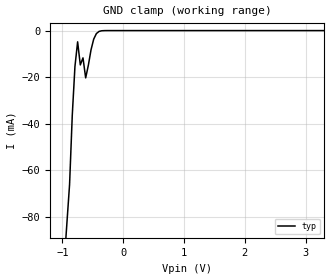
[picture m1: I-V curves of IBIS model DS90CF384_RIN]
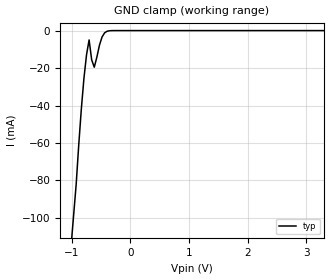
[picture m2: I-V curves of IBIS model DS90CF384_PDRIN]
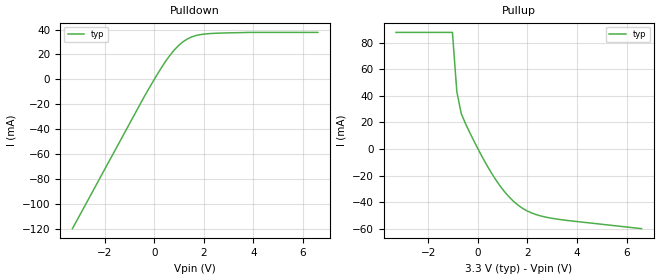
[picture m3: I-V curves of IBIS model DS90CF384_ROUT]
|   National Semiconductor Corporation
|   Interface Products Group
|   IBIS Model of 3.3V FPD-Link Receiver
|   56L TSSOP
[IBIS Ver]   2.1
[File name]   90cf384.ibs
[File Rev]   1.0
[Date]   7/10/98
[Source]   File originated at National Semiconductor Corporation.
   Interface Group/Analog Division. All data based on
   Empirical Measurements(Bench).
[Notes]   File created by SBH.
[Disclaimer]
(C) Copyright National Semiconductor Corporation 1994
   All rights reserved
   National Semiconductor Corporation hereby grants
the user of this IBIS model a non-exclusive, nontransferable
license to use this IBIS model under the following terms.
Before using this IBIS model, the user should read this
license.  If the user does not accept these terms,  the
IBIS model should be returned to National within 30 days.
   The user is granted this license only to use the
IBIS model and is not granted rights to sell, load, rent,
lease or license the IBIS model in whole or in part, or in
modified form to anyone other than user. User may modify
the IBIS model to suit its specific applications but rights
to derivative works and such modifications shall belong to
National.
   This IBIS model is provided on an "AS IS" basis and
National makes absolutely no warranty with respect to the
information contained herein.NATIONAL DISCLAIMS AND CUSTOMER
WAIVES ALL WARRANTIES, EXPRESS OR IMPLIED, INCLUDING
WARRANTIES OF MERCHANTABILITY OR FITNESS FOR A PARTICULAR
PURPOSE. The entire risk as to quality and performance is
with the Customer. ACCORDINGLY, IN NO EVENT SHALL THE
COMPANY BE LIABLE FOR ANY DAMAGES, WHETHER IN CONTRACT OR
TORT,INCLUDING ANY LOST PROFITS OR OTHER INCIDENTAL,
CONSEQUENTIAL, EXEMPLARY, OR PUNITIVE DAMAGES ARISING OUT
OF THE USE OR APPLICATION OF THE IBIS model provided in
this package.Further, National reserves the right to make
changes without notice to any product herein to improve
reliability, function, or design. National does not convey
any license under patent rights or any other intellectual
property rights, including those of third parties.
   National is not obligated to provide maintenance or support
for the licensed IBIS model.
Contact National at ATTN:INTERFACE APPLICATIONS/IBIS MODELS.
2900 Semiconductor Drive, M/S A2595, Santa Clara, CA 95052-8090
[Copyright]   Copyright 1994, National Semiconductor, All Rights Reserved
[Component]   DS90CF384MTD
[Manufacturer]  National Semiconductor Corp
[Package]
|   typ   min   max
R_pkg   35.0m   NA   NA
L_pkg   4.31nH   NA   NA
C_pkg   0.70pF   NA   NA
[Pin]  signal_name   model_name   R_pin   L_pin   C_pin
1   RxOUT22   DS90CF384_ROUT   50.0m   2.07n   0.429p
2   RxOUT23   DS90CF384_ROUT   50.0m   1.49n   0.306p
3   RxOUT24   DS90CF384_ROUT   50.0m   0.95n   0.146p
4   GND   GND   50.0m   0.95n   0.152p
5   RxOUT25   DS90CF384_ROUT   50.0m   0.95n   0.152p
6   RxOUT26   DS90CF384_ROUT   50.0m   0.95n   0.146p
7   RxOUT27   DS90CF384_ROUT   50.0m   1.49n   0.306p
8   LVDSGND   GND   50.0m   2.07n   0.429p
9   RxIN0-   DS90CF384_RIN   50.0m   2.07n   0.429p
10   RxIN0+   DS90CF384_RIN   50.0m   1.49n   0.306p
11   RxIN1-   DS90CF384_RIN   50.0m   0.95n   0.146p
12   RxIN1+   DS90CF384_RIN   50.0m   0.95n   0.152p
13   LVDSVCC   POWER   50.0m   0.95n   0.152p
14   LVDSGND   GND   50.0m   0.95n   0.146p
15   RxIN2-   DS90CF384_RIN   50.0m   1.49n   0.306p
16   RxIN2+   DS90CF384_RIN   50.0m   2.07n   0.429p
17   RxCLKIN-   DS90CF384_RIN   50.0m   2.07n   0.429p
18   RxCLKIN+   DS90CF384_RIN   50.0m   1.49n   0.306p
19   RxIN3-   DS90CF384_RIN   50.0m   0.95n   0.146p
20   RxIN3+   DS90CF384_RIN   50.0m   0.95n   0.152p
21   LVDSGND   GND   50.0m   0.95n   0.152p
22   PLLGND   GND   50.0m   0.95n   0.146p
23   PLLVCC   POWER   50.0m   1.49n   0.306p
24   PLLGND   GND   50.0m   2.07n   0.429p
25   PWRDWN*   DS90CF384_PDRIN   50.0m   2.07n   0.429p
26   RxCLKOUT   DS90CF384_ROUT   50.0m   1.49n   0.306p
27   RxOUT0   DS90CF384_ROUT   50.0m   0.95n   0.146p
28   GND   GND   50.0m   0.95n   0.152p
29   RxOUT1   DS90CF384_ROUT   50.0m   0.95n   0.152p
30   RxOUT2   DS90CF384_ROUT   50.0m   0.95n   0.146p
31   VCC   POWER   50.0m   1.49n   0.306p
32   RxOUT3   DS90CF384_ROUT   50.0m   2.07n   0.429p
33   RxOUT4   DS90CF384_ROUT   50.0m   2.07n   0.429p
34   RxOUT5   DS90CF384_ROUT   50.0m   1.49n   0.306p
35   RxOUT6   DS90CF384_ROUT   50.0m   0.95n   0.146p
36   GND   GND   50.0m   0.95n   0.152p
37   RxOUT7   DS90CF384_ROUT   50.0m   0.95n   0.152p
38   RxOUT8   DS90CF384_ROUT   50.0m   0.95n   0.146p
39   RxOUT9   DS90CF384_ROUT   50.0m   1.49n   0.306p
40   VCC   POWER   50.0m   2.07n   0.429p
41   RxOUT10   DS90CF384_ROUT   50.0m   2.07n   0.429p
42   RxOUT11   DS90CF384_ROUT   50.0m   1.49n   0.306p
43   RxOUT12   DS90CF384_ROUT   50.0m   0.95n   0.146p
44   GND   GND   50.0m   0.95n   0.152p
45   RxOUT13   DS90CF384_ROUT   50.0m   0.95n   0.152p
46   RxOUT14   DS90CF384_ROUT   50.0m   0.95n   0.146p
47   RxOUT15   DS90CF384_ROUT   50.0m   1.49n   0.306p
48   VCC   POWER   50.0m   2.07n   0.429p
49   RxOUT16   DS90CF384_ROUT   50.0m   2.07n   0.429p
50   RxOUT17   DS90CF384_ROUT   50.0m   2.07n   0.429p
51   RxOUT18   DS90CF384_ROUT   50.0m   1.49n   0.306p
52   GND   GND   50.0m   0.95n   0.146p
53   RxOUT19   DS90CF384_ROUT   50.0m   0.95n   0.152p
54   RxOUT20   DS90CF384_ROUT   50.0m   0.95n   0.152p
55   RxOUT21   DS90CF384_ROUT   50.0m   0.95n   0.146p
56   VCC   POWER   50.0m   1.49n   0.306p
[Diff_pin]   inv_pin   vdiff   tdelay_typ   tdelay_min   tdelay_max
| The '+' pin is Diff_pin and the '-' pin is the inv_pin
10   9   0.1   0 0 0
12   11   0.1   0 0 0
16   15   0.1   0 0 0
18   17   0.1   0 0 0
20   19   0.1   0 0 0
| Models and submodels in the file (3): DS90CF384_RIN (Input), DS90CF384_PDRIN (Input), DS90CF384_ROUT (3-state)
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|   RECEIVER INPUT  MODEL
[Model]   DS90CF384_RIN
Model_type   Input
|Signals   RxIN+,RxIN- ; RxCLKIN+, RxCLKIN-
Vinh = 2.0
Vinl = 0.8
|   typ   min   max
C_comp   5.433pF   NA   NA
|   typ   min   max
[Temperature Range]   25.0   NA   NA
[Voltage range]   3.3V   3.0V   3.6V
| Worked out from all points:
|   GND clamp passes 1 mA (typ) near -0.43 V on its own axis
[Power_clamp]
| Note that the[POWER_clamp]voltage table is referenced to Vcc
| and is calculated using Vtable=Vcc - Vmeasured.
|Voltage   I(typ)   I(min)   I(max)
-3V       0A         NA         NA
0V        0A         NA         NA
[GND_clamp]
|Voltage   I(typ)   I(min)   I(max)
-3.3V     -980mA     NA         NA
-882.3mV  -66.02mA   NA         NA
-838.2mV  -36.43mA   NA         NA
-794.1mV  -15.42mA   NA         NA
-750mV    -4.833mA   NA         NA
-705.9mV  -14.74mA   NA         NA
-661.8mV  -11.72mA   NA         NA
-617.7mV  -20.31mA   NA         NA
-485.3mV  -3.653mA   NA         NA
-441.2mV  -1.289mA   NA         NA
-352.9mV  -78.9uA    NA         NA
3.3V      0A         NA         NA
|   RECEIVER PWRDWN* INPUT MODEL
[Model]   DS90CF384_PDRIN
Model_type   Input
|Signals   PWRDWN*
Vinh = 2.0
Vinl = 0.8
|   typ   min   max
C_comp   5.433pF   NA   NA
|   typ   min   max
[Temperature Range]   25.0   NA   NA
[Voltage range]   3.3V   3.0V   3.6V
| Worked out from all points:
|   GND clamp passes 1 mA (typ) near -0.43 V on its own axis
[GND_clamp]
|Voltage   I(typ)   I(min)   I(max)
-3.3V     -980mA     NA         NA
-926.5mV  -82.06mA   NA         NA
-838.2mV  -41.78mA   NA         NA
-794.1mV  -25.51mA   NA         NA
-750mV    -12.98mA   NA         NA
-705.9mV  -4.994mA   NA         NA
-661.8mV  -15.62mA   NA         NA
-617.7mV  -19.54mA   NA         NA
-485.3mV  -3.454mA   NA         NA
-441.2mV  -1.208mA   NA         NA
-352.9mV  -73.7uA    NA         NA
3.3V      0A         NA         NA
[Power_clamp]
| Note that the[POWER_clamp]voltage table is referenced to Vcc
| and is calculated using Vtable=Vcc - Vmeasured.
|Voltage   I(typ)   I(min)   I(max)
-3.3V     0A         0A         0A
0V        0A         0A         0A
|   RECEIVER OUTPUT  MODEL
[Model]   DS90CF384_ROUT
Model_type   3-state
| Signals   RxOUT0 ~ RxOUT20
Vmeas = 1.5V
Cref = 8pF   |Timing specification test load capacitance value
Vref = 0   |Timing specification test load voltage; GND
| variable   typ   min   max
C_comp   5.247pF   NA   NA
|   typ   min   max
[Temperature Range]   25.0   NA   NA
[Voltage range]   3.3V   3.0V   3.6V
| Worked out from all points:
|   slope of the pulldown table from 0 to 0.495 V, typ, clamps not added: 31.7 ohm
|   slope of the pullup table from 0 to 0.495 V, typ, clamps not added: 29.8 ohm
[Pulldown]
| Voltage   I(typ)   I(min)   I(max)
-3.3V     -120mA     NA         NA
-441.2mV  -15.27mA   NA         NA
-88.24mV  -3.072mA   NA         NA
264.7mV   8.581mA    NA         NA
617.6mV   18.91mA    NA         NA
794.1mV   23.29mA    NA         NA
1.147V    30.01mA    NA         NA
1.324V    32.32mA    NA         NA
1.676V    35.18mA    NA         NA
2.206V    36.71mA    NA         NA
3.794V    37.72mA    NA         NA
6.6V      37.72mA    NA         NA
[Pullup]
| Note that the[Pullup]voltage table is referenced to Vcc
| and is calculated using Vtable=Vcc - Vmeasured.
|Voltage   I(typ)   I(min)   I(max)
-3.3V     87.68mA    NA         NA
-1.024V   87.68mA    NA         NA
-847.1mV  43.17mA    NA         NA
-670.6mV  26.7mA     NA         NA
-494.1mV  18.88mA    NA         NA
-141.2mV  5.4mA      NA         NA
564.7mV   -18.56mA   NA         NA
1.094V    -32.6mA    NA         NA
1.624V    -42.33mA   NA         NA
2.153V    -48.04mA   NA         NA
2.859V    -51.77mA   NA         NA
6.6V      -60mA      NA         NA
[GND_clamp]
| Outputs in Tri-state.
| Voltage   I(typ)   I(min)   I(max)
| Receiver output is non-tristable
-3V       0A         NA         NA
3V        0A         NA         NA
[POWER_clamp]
| Note that the[POWER_clamp]voltage table is referenced to Vcc
| and is calculated using Vtable=Vcc - Vmeasured.
| Outputs in Tri-state.
|Voltage   I(typ)   I(min)   I(max)
| Receiver output is non-tristable
-3V       0A         NA         NA
0V        0A         NA         NA
[Ramp]
|   typ   min   max
dV/dt_r   3.3/2.625n   NA   NA
dV/dt_f   3.3/2.654n   NA   NA
R_load = 1MOhm  | Represent Hi-Z
